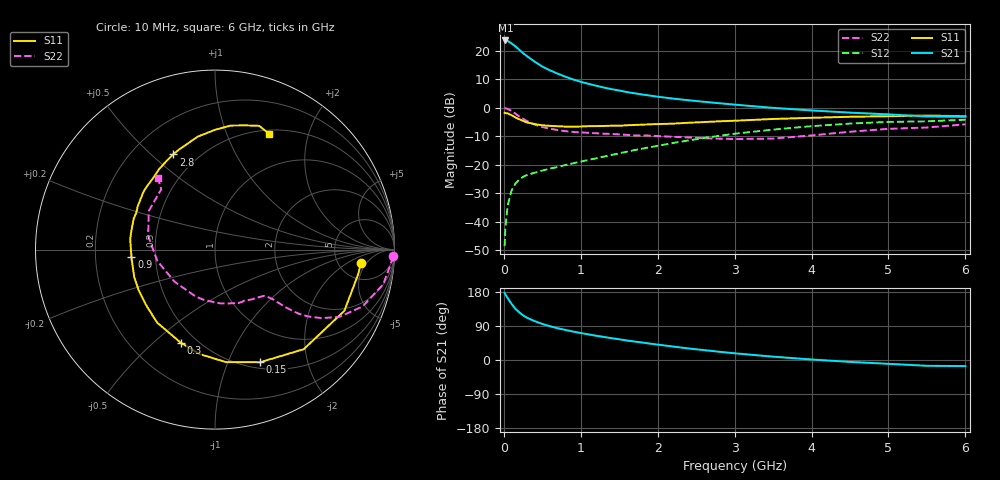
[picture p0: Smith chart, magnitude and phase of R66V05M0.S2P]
! SIEMENS Small Signal Semiconductors
! BFR193
! Si NPN RF Bipolar Junction Transistor in SOT23
! VCE = 6 V  IC = 5 mA
! Common Emitter S-Parameters:  May  1996
# GHz  S  MA  R  50
!  f  S11  S21  S12  S22
! GHz  MAG  ANG  MAG  ANG  MAG  ANG  MAG  ANG
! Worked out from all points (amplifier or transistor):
!   36 points, 10 MHz to 6 GHz, reference 50 ohm
!   highest |S21| = 23.7 dB at 20 MHz (marker M1)
!   |S21| within 3 dB of that: start of sweep to 189 MHz
!   unconditionally stable (mu >= 1): 904.9 MHz to 2.025 GHz
!   at 250 MHz: K = 0.42, MSG = 21.7 dB, |S12| = -24.3 dB
!   at 1.4 GHz: K = 1.06, MAG = 10.1 dB, |S12| = -16.6 dB
!   at 6 GHz: K = 0.96, MSG = 0.5 dB, |S12| = -4.2 dB
!   lowest NFmin = 1.20 dB at 450 MHz
!   S11 on the Smith chart (normalised r, x): 10 MHz: 8.34, -3.65; 150 MHz: 0.57, -1.32; 300 MHz: 0.41, -0.61; 900 MHz: 0.36, -0.04; 2.8 GHz: 0.37, +0.59; 6 GHz: 0.55, +1.43
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0.01  0.8175 -5.1  15.17 176.8  0.0037 90.3  0.9912 -2.2
0.02  0.8087 -10.1  15.28 173.0  0.0077 83.2  0.9822 -4.7
0.05  0.7974 -25.3  14.97 163.1  0.0193 77.3  0.9574 -11.6
0.1  0.7433 -48.3  13.55 148.3  0.035 67.2  0.8819 -21.0
0.15  0.6762 -68.1  12.05 135.1  0.0466 59.1  0.7896 -28.3
0.2  0.6296 -84.5  10.49 125.7  0.0548 54.3  0.7071 -32.7
0.25  0.5884 -98.3  9.132 117.9  0.0612 50.6  0.6404 -35.6
0.3  0.5526 -110.2  8.101 111.6  0.0658 49.1  0.5857 -37.5
0.4  0.519 -128.5  6.493 102.5  0.0724 48.0  0.5065 -39.3
0.5  0.4929 -141.0  5.314 95.2  0.0788 47.9  0.4597 -40.0
0.6  0.4816 -152.2  4.557 89.1  0.0854 48.9  0.43 -40.5
0.7  0.4747 -161.7  3.986 83.8  0.0913 50.6  0.4066 -41.4
0.9  0.4675 -175.2  3.152 75.0  0.1061 53.4  0.3764 -43.3
1.1  0.476 173.0  2.641 67.6  0.1213 56.0  0.3637 -46.6
1.3  0.4797 163.4  2.272 60.8  0.1389 57.8  0.3512 -50.3
1.6  0.4937 150.6  1.893 51.4  0.1695 59.2  0.3342 -57.5
2.2  0.5271 130.8  1.452 35.5  0.2411 57.6  0.3094 -76.0
2.8  0.5793 113.7  1.204 21.8  0.3215 51.8  0.287 -102.2
3.5  0.6367 98.7  0.998 8.8  0.4144 41.2  0.2877 -141.6
4.5  0.6967 82.7  0.823 -5.0  0.5286 24.7  0.3798 168.6
5.5  0.732 70.4  0.704 -15.3  0.5796 7.4  0.4506 131.6
6  0.7124 64.8  0.696 -16.1  0.6182 2.4  0.5129 128.5
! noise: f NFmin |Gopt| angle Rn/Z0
0.45  1.2  0.26  102  0.14
0.9  1.25  0.38  145  0.12
1.8  2.05  0.56  -161  0.12
